| IBIS file stm32u375_385_wlcsp52_smps.ibs
[IBIS ver] 4.2
[File name] stm32u375_385_wlcsp52_smps.ibs
[File Rev] 1.2
[Date] 23-06-2025
[Source] Data Created at STMicroelectronics
[Notes]  File originated from ELDO simulations.
[Disclaimer]  This information is for modeling purpose only and is
   not guaranted. The information is subject to change without
   notice.
[Copyright] Copyright 2025 STMicroelectronics Inc.
|   Component stm32u375_385_wlcsp52_smps
[Component] stm32u375_385_wlcsp52_smps
[Manufacturer] STMicroelectronics
[Package]
| variable   typ   min   max
R_pkg  0  NA  NA
L_pkg  0  NA  NA
C_pkg  0  NA  NA
[Pin]   signal_name   model_name
A1  VDD  power
A3  PA15  io8_ft_100m
A5  PB5  io8_ft_100m_hslv
A7  PB9  io8_ft_100m_hslv
B2  VDDUSB  power
B4  PB3  io8_ft_100m_hslv
B6  PB8  io8_ft_100m_hslv
B8  VDD  power
C1  PA12  io8usb_ft_phy
C3  PA14  io8_ft_100m
C5  PH3-BOOT0  io8_ft_100m_hslv
C7  VSS  gnd
D2  VSS  gnd
D4  PB4  io8_ft_100m_hslv
D6  VBAT  power
D8  PC14-OSC32_IN  io_ft_tamp
E1  PA11  io8usb_ft_phy
E3  PA13  io8_ft_100m
E5  PB7  io8_ft_100m_hslv
E7  PC15-OSC32_OUT  io_ft_tamp
F2  PA10  io8_ft_100m
F4  PB6  io8_ft_100m_hslv
F6  PC13  io8_ft_100m_v33
F8  PH0-OSC_IN  io8_ft_100m
G1  PB15  io8_ft_100m
G3  PA9  io8_ft_100m
G5  PA1  io8_ft_100m_hslv
G7  PH1-OSC_OUT  io8_ft_100m
H2  PA8  io8_ft_100m_hslv
H4  PA2  io8_ft_100m_hslv
H6  PA0  io8_ft_100m
H8  NRST  ioreset_v33
J1  PB14  io8_ft_100m_hslv
J3  PA7  io8_ft_100m_hslv
J5  PA5  io8_ft_100m
J7  VSSA  nc
K2  PB13  io8_ft_100m_hslv
K4  PB0  io8_ft_100m_hslv
K6  PA4  io8_ft_100m_hslv
K8  VDDA  nc
L1  VSS  gnd
L3  VSSSMPS  nc
L5  PB1  io8_ft_100m_hslv
L7  VSS  gnd
M2  VDD11  nc
M4  VLXSMPS  nc
M6  PA6  io8_ft_100m_hslv
M8  PA3  io8_ft_100m_hslv
N1  VDD  power
N3  VDDSMPS  nc
N5  PB2  io8_ft_100m_hslv
N7  VDD  power
[Package Model]   454-wlcsp-52-smps-250423
[Pin Mapping]   pulldown_ref   pullup_ref   | Comment
A1  nc  vddio
A3  gndio  vddio
A5  gndio  vddio
A7  gndio  vddio
B2  nc  vddusb
B4  gndio  vddio
B6  gndio  vddio
B8  nc  vddio
C1  gndio  vddusb  | Depending on IO usage
| C1  gndio  vddio  | Depending on IO usage
C3  gndio  vddio
C5  gndio  vddio
C7  gndio  nc
D2  gndio  nc
D4  gndio  vddio
D6  nc  vsw
D8  gndio  vsw
E1  gndio  vddusb  | Depending on IO usage
| E1  gndio  vddio  | Depending on IO usage
E3  gndio  vddio
E5  gndio  vddio
E7  gndio  vsw
F2  gndio  vddio
F4  gndio  vddio
F6  gndio  vsw
F8  gndio  vddio
G1  gndio  vddio
G3  gndio  vddio
G5  gndio  vddio
G7  gndio  vddio
H2  gndio  vddio
H4  gndio  vddio
H6  gndio  vddio
H8  gndio  vddio
J1  gndio  vddio
J3  gndio  vddio
J5  gndio  vddio
J7  nc  nc
K2  gndio  vddio
K4  gndio  vddio
K6  gndio  vddio
K8  nc  nc
L1  gndio  nc
L3  nc  nc
L5  gndio  vddio
L7  gndio  nc
M2  nc  nc
M4  nc  nc
M6  gndio  vddio
M8  gndio  vddio
N1  nc  vddio
N3  nc  nc
N5  gndio  vddio
N7  nc  vddio
|[Diff Pin]  inv_pin  vdiff  tdelay_typ  tdelay_min  tdelay_max
|C1  E1  NA  NA  NA  NA
[Model Selector] io8_ft_100m
io8_ft_100m_ls_1v2  "GPIO 100MHz - 5V tolerant - low speed - 1.2V range"
io8_ft_100m_ls_1v8  "GPIO 100MHz - 5V tolerant - low speed - 1.8V range"
io8_ft_100m_ls_3v3  "GPIO 100MHz - 5V tolerant - low speed - 3.3V range"
io8_ft_100m_ms_1v2  "GPIO 100MHz - 5V tolerant - med speed - 1.2V range"
io8_ft_100m_ms_1v8  "GPIO 100MHz - 5V tolerant - med speed - 1.8V range"
io8_ft_100m_ms_3v3  "GPIO 100MHz - 5V tolerant - med speed - 3.3V range"
io8_ft_100m_fs_1v2  "GPIO 100MHz - 5V tolerant - fast speed - 1.2V range"
io8_ft_100m_fs_1v8  "GPIO 100MHz - 5V tolerant - fast speed - 1.8V range"
io8_ft_100m_fs_3v3  "GPIO 100MHz - 5V tolerant - fast speed - 3.3V range"
io8_ft_100m_hs_1v2  "GPIO 100MHz - 5V tolerant - high speed - 1.2V range"
io8_ft_100m_hs_1v8  "GPIO 100MHz - 5V tolerant - high speed - 1.8V range"
io8_ft_100m_hs_3v3  "GPIO 100MHz - 5V tolerant - high speed - 3.3V range"
[Model Selector] io8_ft_100m_hslv
io8_ft_100m_ls_1v2  "GPIO 100MHz - 5V tolerant - low speed - 1.2V range"
io8_ft_100m_ls_1v8  "GPIO 100MHz - 5V tolerant - low speed - 1.8V range"
io8_ft_100m_ls_3v3  "GPIO 100MHz - 5V tolerant - low speed - 3.3V range"
io8_ft_100m_ms_1v2  "GPIO 100MHz - 5V tolerant - med speed - 1.2V range"
io8_ft_100m_ms_1v8  "GPIO 100MHz - 5V tolerant - med speed - 1.8V range"
io8_ft_100m_ms_3v3  "GPIO 100MHz - 5V tolerant - med speed - 3.3V range"
io8_ft_100m_fs_1v2  "GPIO 100MHz - 5V tolerant - fast speed - 1.2V range"
io8_ft_100m_fs_1v8  "GPIO 100MHz - 5V tolerant - fast speed - 1.8V range"
io8_ft_100m_fs_3v3  "GPIO 100MHz - 5V tolerant - fast speed - 3.3V range"
io8_ft_100m_hs_1v2  "GPIO 100MHz - 5V tolerant - high speed - 1.2V range"
io8_ft_100m_hs_1v8  "GPIO 100MHz - 5V tolerant - high speed - 1.8V range"
io8_ft_100m_hs_3v3  "GPIO 100MHz - 5V tolerant - high speed - 3.3V range"
io8_ft_100m_hslv_ls_1v2  "GPIO 100MHz low voltage optimization - 5V tolerant - low speed - 1.2V range"
io8_ft_100m_hslv_ls_1v8  "GPIO 100MHz low voltage optimization - 5V tolerant - low speed - 1.8V range"
io8_ft_100m_hslv_ls_2v5  "GPIO 100MHz low voltage optimization - 5V tolerant - low speed - 3.3V range"
io8_ft_100m_hslv_ms_1v2  "GPIO 100MHz low voltage optimization - 5V tolerant - med speed - 1.2V range"
io8_ft_100m_hslv_ms_1v8  "GPIO 100MHz low voltage optimization - 5V tolerant - med speed - 1.8V range"
io8_ft_100m_hslv_ms_2v5  "GPIO 100MHz low voltage optimization - 5V tolerant - med speed - 3.3V range"
io8_ft_100m_hslv_fs_1v2  "GPIO 100MHz low voltage optimization - 5V tolerant - fast speed - 1.2V range"
io8_ft_100m_hslv_fs_1v8  "GPIO 100MHz low voltage optimization - 5V tolerant - fast speed - 1.8V range"
io8_ft_100m_hslv_fs_2v5  "GPIO 100MHz low voltage optimization - 5V tolerant - fast speed - 3.3V range"
io8_ft_100m_hslv_hs_1v2  "GPIO 100MHz low voltage optimization - 5V tolerant - high speed - 1.2V range"
io8_ft_100m_hslv_hs_1v8  "GPIO 100MHz low voltage optimization - 5V tolerant - high speed - 1.8V range"
io8_ft_100m_hslv_hs_2v5  "GPIO 100MHz low voltage optimization - 5V tolerant - high speed - 3.3V range"
[Model Selector] io8_ft_100m_v33
io8_ft_100m_v33_ls_1v2  "GPIO_V33 100MHz - 5V tolerant - low speed - 1.2V range"
io8_ft_100m_v33_ls_1v8  "GPIO_V33 100MHz - 5V tolerant - low speed - 1.8V range"
io8_ft_100m_v33_ls_3v3  "GPIO_V33 100MHz - 5V tolerant - low speed - 3.3V range"
io8_ft_100m_v33_ms_1v2  "GPIO_V33 100MHz - 5V tolerant - med speed - 1.2V range"
io8_ft_100m_v33_ms_1v8  "GPIO_V33 100MHz - 5V tolerant - med speed - 1.8V range"
io8_ft_100m_v33_ms_3v3  "GPIO_V33 100MHz - 5V tolerant - med speed - 3.3V range"
io8_ft_100m_v33_fs_1v2  "GPIO_V33 100MHz - 5V tolerant - fast speed - 1.2V range"
io8_ft_100m_v33_fs_1v8  "GPIO_V33 100MHz - 5V tolerant - fast speed - 1.8V range"
io8_ft_100m_v33_fs_3v3  "GPIO_V33 100MHz - 5V tolerant - fast speed - 3.3V range"
io8_ft_100m_v33_hs_1v2  "GPIO_V33 100MHz - 5V tolerant - high speed - 1.2V range"
io8_ft_100m_v33_hs_1v8  "GPIO_V33 100MHz - 5V tolerant - high speed - 1.8V range"
io8_ft_100m_v33_hs_3v3  "GPIO_V33 100MHz - 5V tolerant - high speed - 3.3V range"
[Model Selector] io8usb_ft_phy
io8_ft_100m_ls_1v2  "GPIO 100MHz - 5V tolerant - low speed - 1.2V range"
io8_ft_100m_ls_1v8  "GPIO 100MHz - 5V tolerant - low speed - 1.8V range"
io8_ft_100m_ls_3v3  "GPIO 100MHz - 5V tolerant - low speed - 3.3V range"
io8_ft_100m_ms_1v2  "GPIO 100MHz - 5V tolerant - med speed - 1.2V range"
io8_ft_100m_ms_1v8  "GPIO 100MHz - 5V tolerant - med speed - 1.8V range"
io8_ft_100m_ms_3v3  "GPIO 100MHz - 5V tolerant - med speed - 3.3V range"
io8_ft_100m_fs_1v2  "GPIO 100MHz - 5V tolerant - fast speed - 1.2V range"
io8_ft_100m_fs_1v8  "GPIO 100MHz - 5V tolerant - fast speed - 1.8V range"
io8_ft_100m_fs_3v3  "GPIO 100MHz - 5V tolerant - fast speed - 3.3V range"
io8_ft_100m_hs_1v2  "GPIO 100MHz - 5V tolerant - high speed - 1.2V range"
io8_ft_100m_hs_1v8  "GPIO 100MHz - 5V tolerant - high speed - 1.8V range"
io8_ft_100m_hs_3v3  "GPIO 100MHz - 5V tolerant - high speed - 3.3V range"
io8usb_ft_phy_hs_3v3   "USB full speed"
io8usb_ft_phy_ls_3v3   "USB low speed"
[Model Selector] io_ft_tamp
io_ft_tamp_ls_1v2 "io8_ft tamp low speed @ 1.2V"
io_ft_tamp_ls_1v8 "io8_ft tamp low speed @ 1.8V"
io_ft_tamp_ls_3v3 "io8_ft tamp low speed @ 3.3V"
io_ft_tamp_ms_1v2 "io8_ft tamp med speed @ 1.2V"
io_ft_tamp_ms_1v8 "io8_ft tamp med speed @ 1.8V"
io_ft_tamp_ms_3v3 "io8_ft tamp med speed @ 3.3V"
io_ft_tamp_fs_1v2 "io8_ft tamp fast speed @ 1.2V"
io_ft_tamp_fs_1v8 "io8_ft tamp fast speed @ 1.8V"
io_ft_tamp_fs_3v3 "io8_ft tamp fast speed @ 3.3V"
io_ft_tamp_hs_1v2 "io8_ft tamp high speed @ 1.2V"
io_ft_tamp_hs_1v8 "io8_ft tamp high speed @ 1.8V"
io_ft_tamp_hs_3v3 "io8_ft tamp high speed @ 3.3V"
[Model Selector] ioreset_v33
ioreset_v33_1v2 "Reset PAD. 5V tolerant. 1.2V range"
ioreset_v33_1v8 "Reset PAD. 5V tolerant. 1.8V range"
ioreset_v33_3v3 "Reset PAD. 5V tolerant. 3.3V range"
[Define Package Model]  454-wlcsp-52-smps-250423
[Manufacturer]  Unknown
[OEM]  Unknown
[Description]  None
[Number Of Pins]  49
[Pin Numbers]
| Pin Num   Terminal Name
H8 | NRST
H6 | PA0
G5 | PA1
H4 | PA2
M8 | PA3
K6 | PA4
J5 | PA5
M6 | PA6
J3 | PA7
H2 | PA8
G3 | PA9
F2 | PA10
E1 | PA11
C1 | PA12
E3 | PA13
C3 | PA14
A3 | PA15
K4 | PB0
L5 | PB1
N5 | PB2
B4 | PB3
D4 | PB4
A5 | PB5
F4 | PB6
E5 | PB7
B6 | PB8
A7 | PB9
K2 | PB13
J1 | PB14
G1 | PB15
F6 | PC13
D8 | PC14-OSC32_IN
E7 | PC15-OSC32_OUT
F8 | PH0-OSC_IN
G7 | PH1-OSC_OUT
C5 | PH3-BOOT0
M2 | VDD11
D6 | VBAT
A1 | VDD
B8 | VDD
N1 | VDD
N7 | VDD
K8 | VDDA
N3 | VDDSMPS
B2 | VDDUSB
M4 | VLXSMPS
C7 | VSS
J7 | VSSA
L3 | VSSSMPS
|[Merged Pins]  C7
|D2  |  VSS
|L1  |  VSS
|L7  |  VSS
[Model Data]
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[End Model Data]
[End Package Model]
|End [Component]
| Models and submodels in the file (53): io8_ft_100m_fs_1v2 (I/O), io8_ft_100m_fs_1v8 (I/O), io8_ft_100m_fs_3v3 (I/O), io8_ft_100m_hs_1v2 (I/O), io8_ft_100m_hs_1v8 (I/O), io8_ft_100m_hs_3v3 (I/O), io8_ft_100m_hslv_fs_1v2 (I/O), io8_ft_100m_hslv_fs_1v8 (I/O), io8_ft_100m_hslv_fs_2v5 (I/O), io8_ft_100m_hslv_hs_1v2 (I/O), io8_ft_100m_hslv_hs_1v8 (I/O), io8_ft_100m_hslv_hs_2v5 (I/O), io8_ft_100m_hslv_ls_1v2 (I/O), io8_ft_100m_hslv_ls_1v8 (I/O), io8_ft_100m_hslv_ls_2v5 (I/O), io8_ft_100m_hslv_ms_1v2 (I/O), io8_ft_100m_hslv_ms_1v8 (I/O), io8_ft_100m_hslv_ms_2v5 (I/O), io8_ft_100m_ls_1v2 (I/O), io8_ft_100m_ls_1v8 (I/O), io8_ft_100m_ls_3v3 (I/O), io8_ft_100m_ms_1v2 (I/O), io8_ft_100m_ms_1v8 (I/O), io8_ft_100m_ms_3v3 (I/O), io8_ft_100m_v33_fs_1v2 (I/O), io8_ft_100m_v33_fs_1v8 (I/O), io8_ft_100m_v33_fs_3v3 (I/O), io8_ft_100m_v33_hs_1v2 (I/O), io8_ft_100m_v33_hs_1v8 (I/O), io8_ft_100m_v33_hs_3v3 (I/O), io8_ft_100m_v33_ls_1v2 (I/O), io8_ft_100m_v33_ls_1v8 (I/O), io8_ft_100m_v33_ls_3v3 (I/O), io8_ft_100m_v33_ms_1v2 (I/O), io8_ft_100m_v33_ms_1v8 (I/O), io8_ft_100m_v33_ms_3v3 (I/O), io8usb_ft_phy_hs_3v3 (I/O), io8usb_ft_phy_ls_3v3 (I/O), io_ft_tamp_fs_1v2 (I/O), io_ft_tamp_fs_1v8 (I/O), io_ft_tamp_fs_3v3 (I/O), io_ft_tamp_hs_1v2 (I/O), io_ft_tamp_hs_1v8 (I/O), io_ft_tamp_hs_3v3 (I/O), io_ft_tamp_ls_1v2 (I/O), io_ft_tamp_ls_1v8 (I/O), io_ft_tamp_ls_3v3 (I/O), io_ft_tamp_ms_1v2 (I/O), io_ft_tamp_ms_1v8 (I/O), io_ft_tamp_ms_3v3 (I/O), ioreset_v33_1v2 (I/O_open_drain), ioreset_v33_1v8 (I/O_open_drain), ioreset_v33_3v3 (I/O_open_drain)
